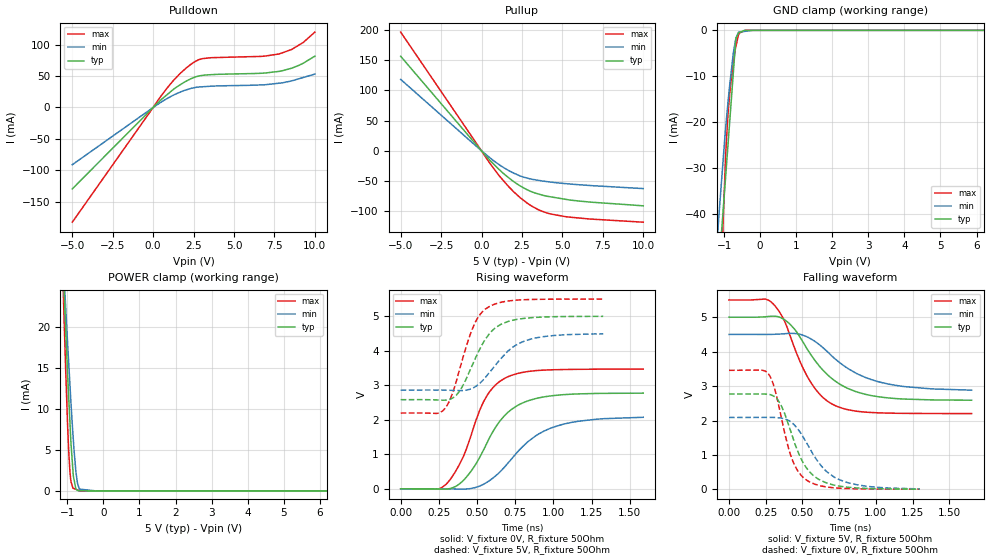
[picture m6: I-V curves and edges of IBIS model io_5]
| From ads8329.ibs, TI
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|   io_5 Model
[Model]   io_5
Model_type   I/O
Polarity   Non-Inverting
Enable   Active-Low
Vinl = 1.75
Vinh = 3.25
Vmeas = 2.5
Vref = 2.5
Cref = 30pF
Rref = 50
|   typ   min   max
|   (nom PVT)   (Fast PVT)   (slow PVT)
|C_comp from frequency sweep method(F=50MHz)
C_comp   3.642e-12   3.510e-12   3.791e-12
|ON state : BUFFER OUTPUT TURNED HIGH
|C_comp   3.984e-12   3.870e-12   4.164e-12
|OFF state: BUFFER OUTPUT TURNED LOW
|C_comp   3.642e-12   3.510e-12   3.791e-12
|C_comp from LC tank measurement(L=1nH)
|C_comp   2.9805e-12  2.730e-12   3.131e-12
|OFF state: BUFFER OUTPUT TURNED LOW
|Resonant Frequency(Hz)   3.000e+09   3.120e+09   2.940e+09
|C_comp   2.817e-12   2.605e-12   2.933e-12
|ON state : BUFFER OUTPUT TURNED HIGH
|Resonant Frequency(Hz)   2.840e+09   2.980e+09   2.760e+09
|C_comp   3.144e-12   2.855e-12   3.329e-12
| Where nom  PVT is Nominal Process,  5V,  28C
|   Fast PVT is Strong Process,   5.5V,  -40C
|   Slow PVT is Weak Process,   4.5V,  88C
[Model Spec]
Vinl   1.75   1.57   1.92
Vinh   3.25   2.92   3.57
[Voltage Range]   5   4.5   5.5
|Ambient Temperature   25   85   -40
|Junction Temperature
[Temperature Range]   28   88   -40
[Pullup Reference]   5   4.5   5.5
[Pulldown Reference]   0   0   0
[Power Clamp Reference]   5   4.5   5.5
[GND Clamp Reference]   0   0   0
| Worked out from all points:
|   slope of the pulldown table from 0 to 0.75 V, typ, clamps not added: 41.6 ohm
|   slope of the pullup table from 0 to 0.75 V, typ, clamps not added: 34.4 ohm
|   GND clamp passes 1 mA (typ) near -0.63 V on its own axis
|   POWER clamp passes 1 mA (typ) near -0.80 V on its own axis
|   falling waveform, V_fixture 5V, R_fixture 50Ohm: 20-80 % time 280ps typ, 335ps min, 215ps max; typ from 5 V to 2.59 V
|   rising waveform, V_fixture 0V, R_fixture 50Ohm: 20-80 % time 235ps typ, 300ps min, 193ps max; typ from 0 V to 2.77 V
|   rising waveform, V_fixture 5V, R_fixture 50Ohm: 20-80 % time 169ps typ, 209ps min, 144ps max; typ from 2.58 V to 5 V
|   falling waveform, V_fixture 0V, R_fixture 50Ohm: 20-80 % time 162ps typ, 211ps min, 127ps max; typ from 2.77 V to 0.008 V
[Pulldown]
|   Voltage   I(typ)   I(min)   I(max)
-5V       -129.7mA   -91.16mA   -182.7mA
544.5mV   13.56mA    9.392mA    20.29mA
1.27V     29.15mA    19.86mA    43.43mA
2.084V    42.51mA    28.38mA    63.78mA
2.574V    48.25mA    31.78mA    72.91mA
3.08V     51.29mA    33.04mA    77.94mA
6.6V      54.42mA    35.87mA    81.3mA
7.788V    57.5mA     38.68mA    85.29mA
8.563V    62.61mA    42.36mA    92.36mA
9.28V     70.47mA    47.78mA    103.6mA
10V       81.79mA    53.22mA    120.1mA
[GND Clamp]
|   Voltage   I(typ)   I(min)   I(max)
-5V       -897.3mA   -658.7mA   -1.295A
-1.238V   -68.2mA    -51.34mA   -96.17mA
-1.143V   -51.64mA   -40.1mA    -70.51mA
-1.028V   -39.31mA   -28.37mA   -41.82mA
-957mV    -31.74mA   -21.13mA   -27.29mA
-891mV    -24.74mA   -15.56mA   -18.12mA
-814mV    -16.59mA   -9.738mA   -11.5mA
-742.5mV  -9.016mA   -4.846mA   -6.946mA
-675mV    -1.867mA   -1.787mA   -3.58mA
-598.5mV  -555.5uA   -394.5uA   -973.7uA
-407mV    -7.391uA   -203.8uA   -2.213uA
10V       0A         0A         0A
[Pullup]
|   Voltage   I(typ)   I(min)   I(max)
-5V       156.7mA    118.4mA    196.7mA
456.5mV   -13.76mA   -9.979mA   -18.22mA
1.166V    -32.83mA   -24.21mA   -43.49mA
1.672V    -44.32mA   -32.44mA   -59.07mA
2.376V    -57.83mA   -41.4mA    -77.2mA
3.08V     -67.48mA   -46.84mA   -91.12mA
3.526V    -71.47mA   -48.82mA   -97.64mA
4.268V    -76.1mA    -51.66mA   -104.5mA
5.192V    -80.22mA   -54.24mA   -109mA
6.6V      -84.52mA   -57.17mA   -112.6mA
10V       -91.03mA   -62.47mA   -118.1mA
[POWER Clamp]
|   Voltage   I(typ)   I(min)   I(max)
-5V       207.8mA    188.7mA    235.2mA
-1.14V    29.99mA    30.26mA    28.19mA
-1.105V   26.12mA    27.21mA    23.03mA
-1.098V   25.28mA    26.55mA    21.95mA
-1.045V   19.51mA    22.19mA    14.5mA
-990mV    13.86mA    17.67mA    7.634mA
-929.5mV  8.415mA    12.99mA    2.38mA
-835mV    1.831mA    6.223mA    318.2uA
-720mV    60.44uA    951.4uA    122.3uA
-666mV    12.23uA    221.7uA    30.32uA
-202.5mV  0A         0A         427.1nA
10V       0A         0A         0A
[Ramp]
R_load = 50
|   typ   min   max
dV/dt_r   1.66606/2.35835e-10   1.25382/3.05392e-10   2.08305/1.93571e-10
dV/dt_f   1.44971/2.80879e-10   0.982052/3.4346e-10   1.98119/2.15332e-10
[Falling Waveform]
V_fixture = 5V
V_fixture_min = 4.5V
V_fixture_max = 5.5V
R_fixture = 50Ohm
|   Time   V(typ)   V(min)   V(max)
0s        5V         4.5V       5.5V
248ps     5.012V     4.499V     5.527V
298ps     5.029V     4.502V     5.398V
368ps     4.953V     4.517V     4.972V
420ps     4.775V     4.532V     4.411V
550ps     3.958V     4.389V     3.154V
632ps     3.497V     4.143V     2.699V
724ps     3.141V     3.784V     2.431V
1.044ns   2.675V     3.097V     2.219V
1.652ns   2.589V     2.881V     2.201V
[Rising Waveform]
V_fixture = 0V
V_fixture_min = 0V
V_fixture_max = 0V
R_fixture = 50Ohm
|   Time   V(typ)   V(min)   V(max)
0s        1.719nV    1.915nV    1.479nV
242ps     -3.637mV   628uV      -5.3mV
302ps     -5.598mV   -960.2uV   152.7mV
412ps     251.1mV    -9.911mV   952.7mV
548ps     1.173V     145.5mV    2.566V
606ps     1.672V     318.1mV    2.94V
680ps     2.119V     629.9mV    3.198V
836ps     2.553V     1.376V     3.4V
1ns       2.701V     1.787V     3.449V
1.588ns   2.771V     2.072V     3.469V
[Rising Waveform]
V_fixture = 5V
V_fixture_min = 4.5V
V_fixture_max = 5.5V
R_fixture = 50Ohm
|   Time   V(typ)   V(min)   V(max)
0s        2.582V     2.861V     2.196V
236ps     2.575V     2.861V     2.185V
288ps     2.567V     2.858V     2.318V
328ps     2.601V     2.853V     2.634V
378ps     2.784V     2.847V     3.338V
480ps     3.691V     2.935V     4.743V
580ps     4.488V     3.364V     5.278V
706ps     4.851V     4.003V     5.442V
814ps     4.941V     4.288V     5.479V
1.326ns   4.996V     4.492V     5.497V
[Falling Waveform]
V_fixture = 0V
V_fixture_min = 0V
V_fixture_max = 0V
R_fixture = 50Ohm
|   Time   V(typ)   V(min)   V(max)
0s        2.769V     2.088V     3.457V
274ps     2.757V     2.09V      3.32V
308ps     2.698V     2.088V     2.964V
350ps     2.478V     2.073V     2.213V
420ps     1.691V     1.964V     988.2mV
468ps     1.109V     1.755V     538.8mV
530ps     609.7mV    1.337V     263.9mV
630ps     249.7mV    672.1mV    96.97mV
752ps     94.3mV     280.5mV    34mV
1.298ns   7.67mV     14.01mV    6.314mV
